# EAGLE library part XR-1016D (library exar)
Seventh order switched capacitor FILTER
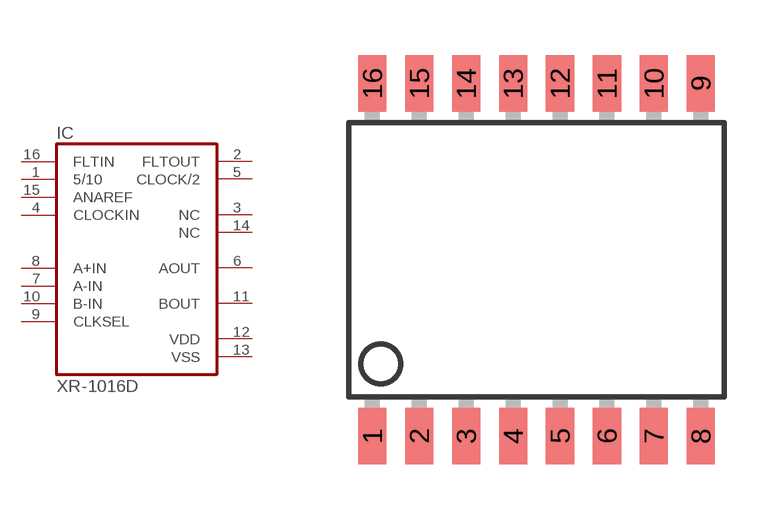
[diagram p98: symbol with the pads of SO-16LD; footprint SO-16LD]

Designator prefix IC

## XR-1016D (OC_FARNELL: unknown; OC_NEWARK: unknown)  [SO-16LD]
1  5/10  in
2  FLTOUT  out
3  NC  nc
4  CLOCKIN  in
5  CLOCK/2  out
6  AOUT  out
7  A-IN  in
8  A+IN  in
9  CLKSEL  in
10  B-IN  in
11  BOUT  out
12  VDD  pwr
13  VSS  pwr
14  NC  nc
15  ANAREF  in
16  FLTIN  in

## Footprint SO-16LD (pad centres in mm)
Small Outline Package
smd 0.762 x 1.524: 1 -4.445,-4.775; 2 -3.175,-4.775; 3 -1.905,-4.775; 4 -0.635,-4.775; 5 0.635,-4.775; 6 1.905,-4.775; 7 3.175,-4.775; 8 4.445,-4.775; 9 4.445,4.775; 10 3.175,4.775; 11 1.905,4.775; 12 0.635,4.775; 13 -0.635,4.775; 14 -1.905,4.775; 15 -3.175,4.775; 16 -4.445,4.775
